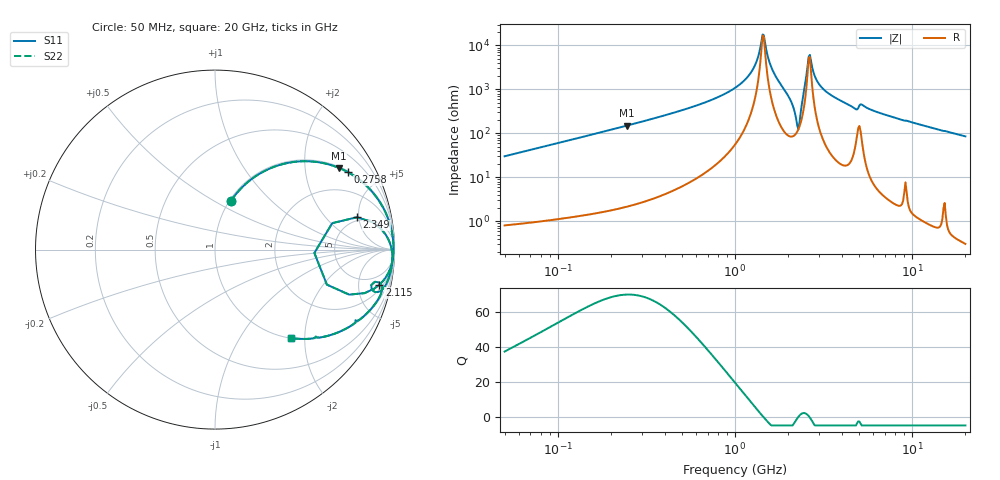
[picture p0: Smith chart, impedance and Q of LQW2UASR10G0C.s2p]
!Murata Part Number: LQW2UASR10G0C
!These Parameters are Measured in Series Mode Connection
!  o--[Z]--o
!Port1  Port2
!  o-------o
!Freq. Start=50[MHz] Stop=20[GHz], 401[Steps]
# Hz S RI R 50
!Freq.(Hz) S11(Real) S11(Imag) S21(Real) S21(Imag) S12(Real) S12(Imag) S22(Real) S22(Imag)
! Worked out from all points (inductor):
!   401 points, 50 MHz to 20 GHz, reference 50 ohm
!   read as one part in series: L = 95.8 nH near 51.52 MHz
!   highest Q = 69.9 at 244.6 MHz (marker M1), where L = 97.7 nH
!   self-resonance near 1.433 GHz
!   S11 on the Smith chart (normalised r, x): 50 MHz: 1.02, +0.60; 275.8 MHz: 1.05, +3.41; 2.115 GHz: 2.71, -8.62; 2.349 GHz: 4.49, +4.74; 20 GHz: 1.01, -1.71
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5e7  0.0897 0.2726  0.9103 -0.2726  0.9103 -0.2726  0.0897 0.2726
1.364002e8  0.406 0.483  0.594 -0.483  0.594 -0.483  0.406 0.483
2.446335e8  0.6903 0.4553  0.3097 -0.4553  0.3097 -0.4553  0.6903 0.4553
2.757764e8  0.741 0.431  0.259 -0.431  0.259 -0.431  0.741 0.431
3.721004e8  0.8446 0.3547  0.1554 -0.3547  0.1554 -0.3547  0.8446 0.3547
1e9  0.987 0.0905  0.013 -0.0905  0.013 -0.0905  0.987 0.0905
1.251922e9  0.9938 0.0362  0.0062 -0.0362  0.0062 -0.0362  0.9938 0.0362
1.329223e9  0.9945 0.0212  0.00547 -0.0212  0.00547 -0.0212  0.9945 0.0212
1.411297e9  0.9948 0.00579  0.00525 -0.00579  0.00525 -0.00579  0.9948 0.00579
1.454215e9  0.9946 -0.0022  0.00535 0.0022  0.00535 0.0022  0.9946 -0.0022
1.639343e9  0.9923 -0.0372  0.00771 0.0372  0.00771 0.0372  0.9923 -0.0372
2.114743e9  0.9158 -0.1957  0.0842 0.1957  0.0842 0.1957  0.9158 -0.1957
2.245319e9  0.6235 -0.1952  0.3765 0.1952  0.3765 0.1952  0.6235 -0.1952
2.348516e9  0.7912 0.1803  0.2088 -0.1803  0.2088 -0.1803  0.7912 0.1803
2.608132e9  0.9832 0.00567  0.0168 -0.00567  0.0168 -0.00567  0.9832 0.00567
2.728004e9  0.9878 -0.0284  0.0122 0.0284  0.0122 0.0284  0.9878 -0.0284
2.98453e9  0.9869 -0.074  0.0131 0.074  0.0131 0.074  0.9869 -0.074
3.519108e9  0.9757 -0.1337  0.0243 0.1337  0.0243 0.1337  0.9757 -0.1337
4.748272e9  0.9063 -0.2368  0.0937 0.2368  0.0937 0.2368  0.9063 -0.2368
5.194772e9  0.925 -0.1949  0.075 0.1949  0.075 0.1949  0.925 -0.1949
7.442007e9  0.8576 -0.3435  0.1424 0.3435  0.1424 0.3435  0.8576 -0.3435
2e10  0.4237 -0.4924  0.5763 0.4924  0.5763 0.4924  0.4237 -0.4924
